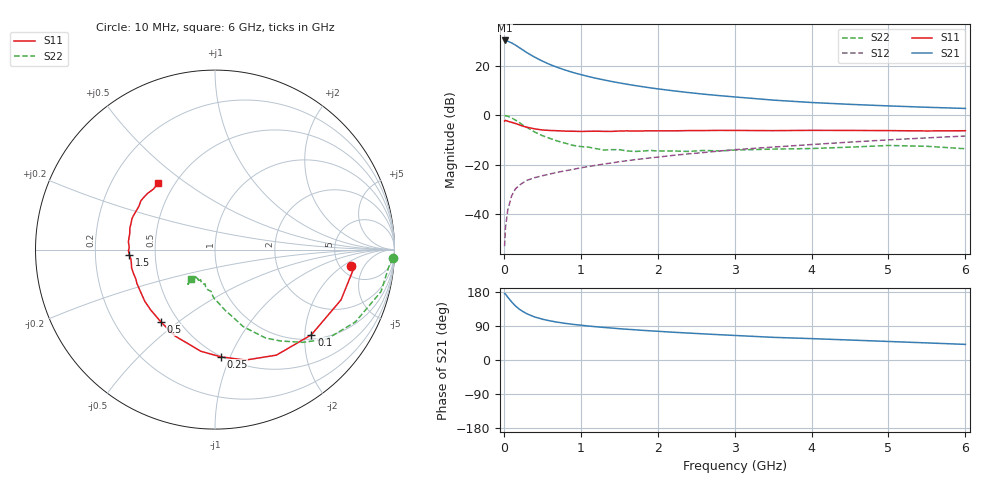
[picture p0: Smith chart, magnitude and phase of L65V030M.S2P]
!  INFINEON TECHNOLOGIES Small Signal Semiconductors
! BFR380L3 , Si-NPN RF-Transistor in TSLP-3-1
!  Vce=5 V,  Ic=30 mA
! Common Emitter S-Parameters:  07. March 2005
#  GHz  S  MA  R  50
! f  S11  S21  S12  S22
! GHz  Mag  Ang  Mag  Ang  Mag  Ang  Mag  Ang
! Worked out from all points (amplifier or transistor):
!   36 points, 10 MHz to 6 GHz, reference 50 ohm
!   highest |S21| = 30.1 dB at 10 MHz (marker M1)
!   |S21| within 3 dB of that: start of sweep to 205.9 MHz
!   unconditionally stable (mu >= 1): 1.995 GHz to 4.772 GHz
!   at 250 MHz: K = 0.36, MSG = 26.7 dB, |S12| = -27.2 dB
!   at 1.4 GHz: K = 0.94, MSG = 16.4 dB, |S12| = -19.3 dB
!   at 6 GHz: K = 0.97, MSG = 5.5 dB, |S12| = -8.4 dB
!   S11 on the Smith chart (normalised r, x): 10 MHz: 6.22, -2.61; 100 MHz: 1.10, -2.16; 250 MHz: 0.50, -0.92; 500 MHz: 0.40, -0.43; 1.5 GHz: 0.35, -0.03; 6 GHz: 0.41, +0.40
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0.01  0.7602 -6.7  31.95 175.1  0.0023 70.7  0.9921 -2.7
0.02  0.7863 -6.0  31.76 174.4  0.0052 90.6  0.9723 -5.8
0.05  0.7561 -21.7  30.92 165.9  0.012 81.1  0.9542 -14.2
0.1  0.7168 -41.5  28.56 153.6  0.0235 71.1  0.8802 -27.2
0.15  0.6803 -59.8  25.83 142.8  0.0326 65.0  0.7983 -38.6
0.2  0.6387 -74.5  22.93 134.3  0.0388 60.2  0.7113 -46.6
0.25  0.5984 -86.9  20.42 127.7  0.0436 56.3  0.627 -54.3
0.3  0.572 -97.9  18.15 121.9  0.0487 55.2  0.5678 -60.2
0.4  0.5305 -114.7  14.75 113.6  0.055 52.5  0.4582 -69.8
0.5  0.5031 -126.9  12.29 107.8  0.0602 53.0  0.3875 -75.3
0.6  0.4914 -136.7  10.46 103.2  0.0654 53.0  0.3397 -80.9
0.7  0.4858 -143.6  9.126 99.7  0.0709 54.5  0.3002 -85.9
0.9  0.4743 -156.5  7.223 94.0  0.0809 56.3  0.2464 -94.4
1.1  0.4732 -163.9  5.999 89.6  0.0924 58.1  0.2272 -100.1
1.5  0.4783 -176.4  4.471 82.6  0.1155 60.9  0.2019 -110.2
1.9  0.4844 174.9  3.556 77.0  0.1377 62.2  0.1949 -118.9
2.2  0.4833 169.4  3.099 73.3  0.1548 62.6  0.1901 -119.8
2.8  0.4937 159.5  2.475 66.8  0.1893 63.4  0.1902 -127.3
3.5  0.4878 150.4  2.01 59.8  0.2276 62.0  0.2073 -127.6
4.5  0.4924 144.0  1.651 52.7  0.2869 61.2  0.2269 -128.1
5.5  0.4812 135.7  1.442 45.1  0.3486 58.1  0.236 -128.0
6  0.4859 130.5  1.365 41.2  0.3805 56.2  0.2107 -129.2
